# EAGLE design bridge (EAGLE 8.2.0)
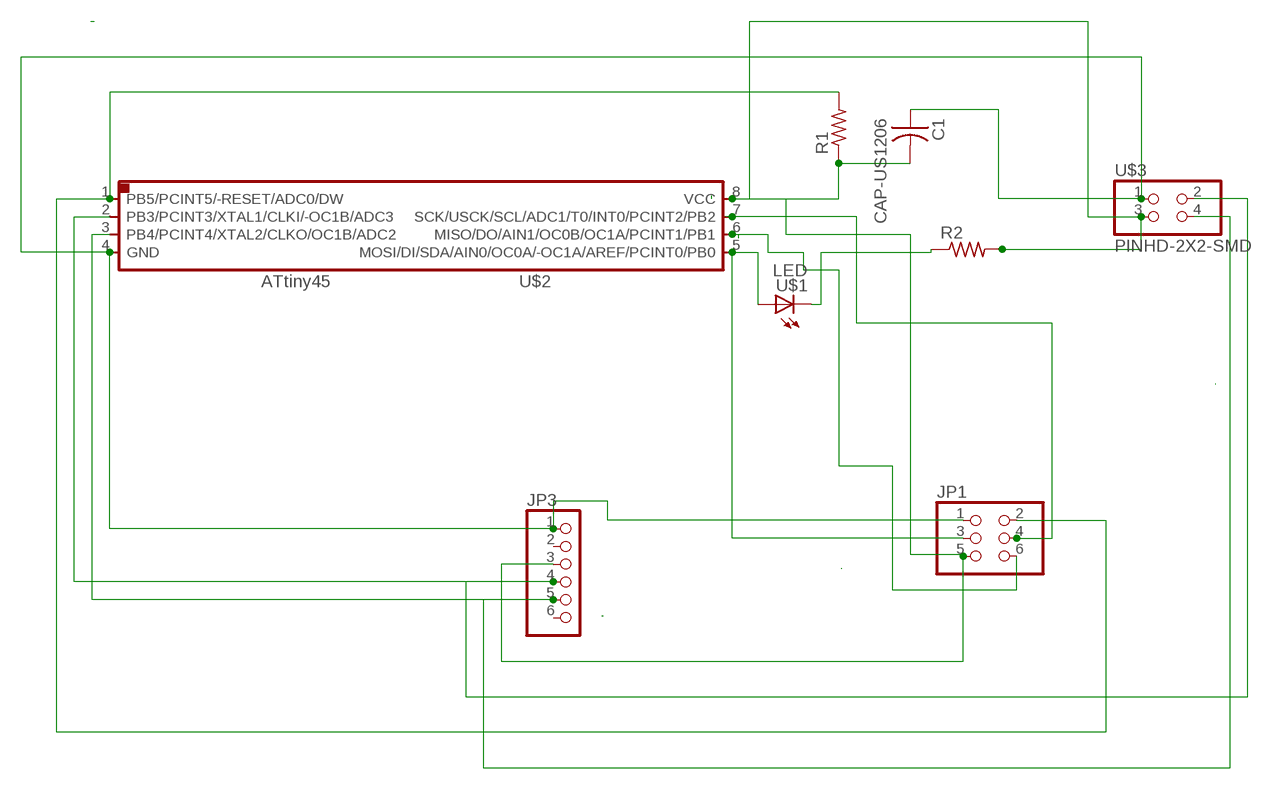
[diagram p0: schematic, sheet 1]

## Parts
C1  CAP-US1206  [C1206]
JP1  PINHD-2X3-SMD  [2X03SMD]
JP3  PINHD-1X6  [1X06]
R1  RES-US1206  [R1206]
R2  RES-US1206  [R1206]
U$1  LED  [LED1206]
U$2  ATTINY45SI  [SOIC8]
U$3  PINHD-2X2-SMD  [2X02SMD]

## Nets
N$2: JP1.6 U$2.6(MISO/DO/AIN1/OC0B/OC1A/PCINT1/PB1)
N$4: C1.1 JP1.1 JP3.1 U$2.4(GND) U$3.1
N$5: JP1.4 U$2.7(SCK/USCK/SCL/ADC1/T0/INT0/PCINT2/PB2)
N$6: JP3.4 U$2.2(PB3/PCINT3/XTAL1/CLKI/-OC1B/ADC3) U$3.2
N$7: JP3.5 U$2.3(PB4/PCINT4/XTAL2/CLKO/OC1B/ADC2) U$3.4
N$9: R2.1 U$1.2(C)
N$10: JP1.3 U$1.1(A) U$2.5(MOSI/DI/SDA/AIN0/OC0A/-OC1A/AREF/PCINT0/PB0)
N$12: JP1.2 R1.2 U$2.1(PB5/PCINT5/-RESET/ADC0/DW)
N$22: C1.2 JP1.5 JP3.3 R1.1 R2.2 U$2.8(VCC) U$3.3
Unconnected: JP3.2 JP3.6

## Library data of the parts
C1 = fab:CAP-US
JP1 = fab:PINHD-2X3-SMD: PIN HEADER
JP3 = pinhead:PINHD-1X6: PIN HEADER
R1 R2 = fab:RES-US: Resistor (US Symbol)
U$1 = fab:LED: LED
U$2 = fab:ATTINY45
U$3 = fab:PINHD-2X2-SMD

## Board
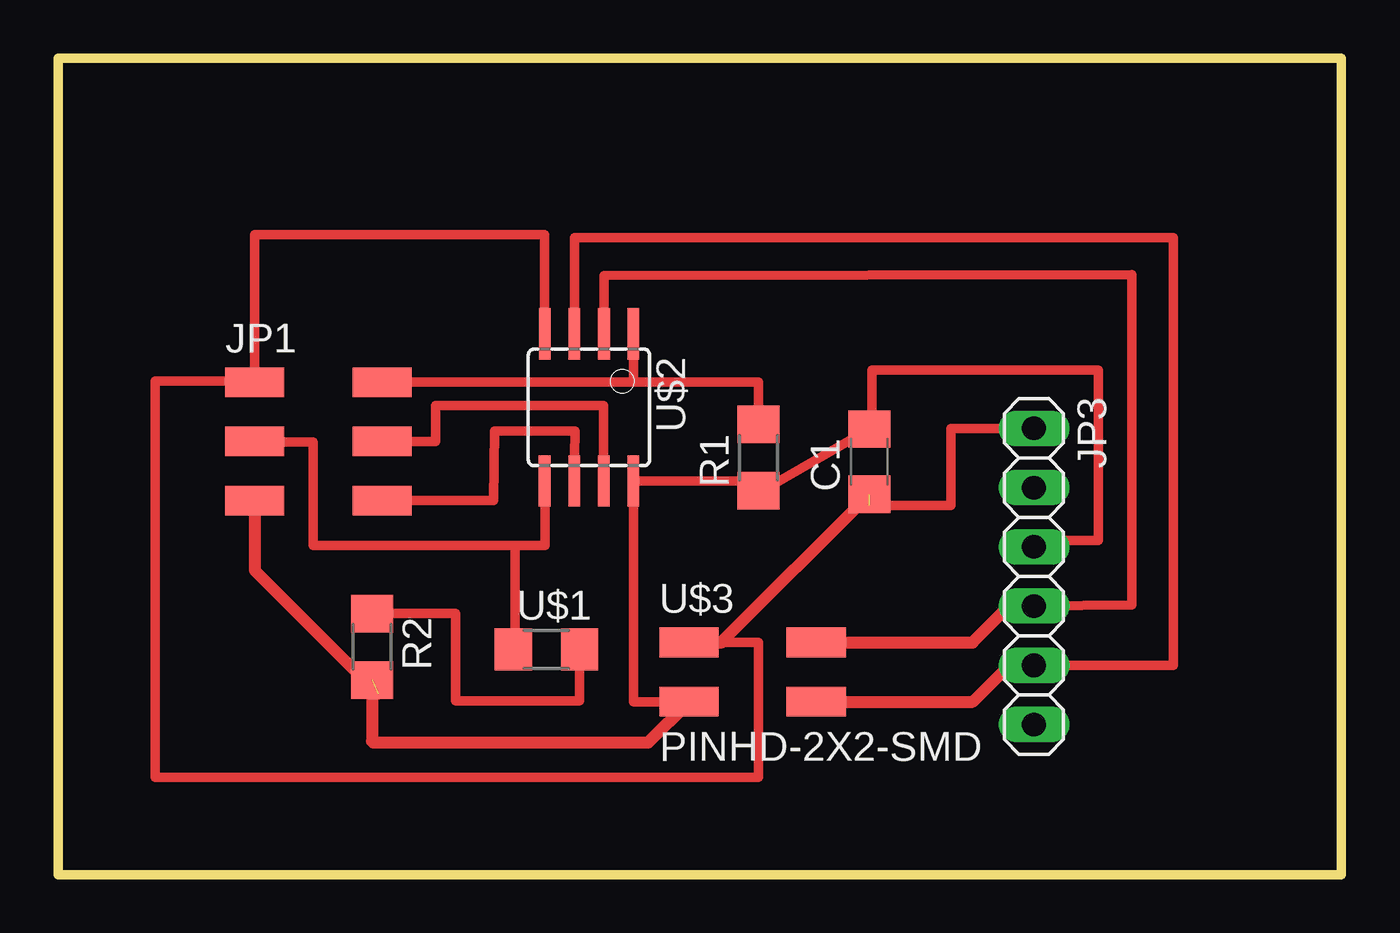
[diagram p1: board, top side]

Size 55 x 35 mm. Coordinates in mm from the lower left corner, seen from the top.
Outline: 0,35 0,0 55,0 55,35 0,35
Copper layers (1*16): Top 0.035mm / dielectric 1.5mm / Bottom 0.035mm
Design rules "default": minimum track width 10mil, minimum drill 24mil, track to track 8mil, track to pad 8mil, pad to pad 8mil, via to via 8mil, smd to smd 8mil, copper to edge 40mil, drill to drill 8mil, minimum pad ring 10mil, minimum via ring 8mil, stop-mask expansion 4mil, vias tented up to drill 0mil, thermal gap 10mil

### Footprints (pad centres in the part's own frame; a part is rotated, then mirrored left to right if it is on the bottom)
C1206 = smd 1.6 x 1.8: 1 -1.4,0; 2 1.4,0
2X03SMD = smd 2.54 x 1.27: 1 -2.54,2.54; 2 2.92,2.54; 3 -2.54,0; 4 2.92,0; 5 -2.54,-2.54; 6 2.92,-2.54
1X06 = drill 1.016 long: 1 -6.35,0; 2 -3.81,0; 3 -1.27,0; 4 1.27,0; 5 3.81,0; 6 6.35,0
R1206 = smd 1.6 x 1.803: 1 -1.422,0; 2 1.422,0
LED1206 = smd 1.6 x 1.803: 1 -1.422,0; 2 1.422,0
SOIC8 = smd 0.5 x 2.2: 1 -1.905,-3.154; 2 -0.645,-3.154; 3 0.625,-3.154; 4 1.895,-3.154; 5 1.905,3.154; 6 0.635,3.154; 7 -0.635,3.154; 8 -1.905,3.154
2X02SMD = smd 2.54 x 1.27: 1 -2.54,1.27; 2 2.92,1.27; 3 -2.54,-1.27; 4 2.92,-1.27

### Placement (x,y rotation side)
C1  34.77,17.7 90 top
JP1  10.96,18.57 0 top
JP3  41.83,12.78 270 top
R1  30.02,17.88 90 top
R2  13.45,9.76 270 top
U$1  20.92,9.66 0 top
U$2  22.75,20.03 180 top
U$3  29.58,8.68 0 top

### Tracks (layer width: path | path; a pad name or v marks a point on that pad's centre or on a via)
N$2
  Top 0.406: JP1.6 18.67,16.03 18.71,19.02 22.16,19.02 U$2.6
N$4  (1 unrouted)
  Top 0.406: U$2.4 20.86,27.44 8.42,27.44 8.42,24.39 JP1.1 8.42,21.17 4.15,21.17 4.15,4.16 30.02,4.16 30.02,9.95 U$3.1 | JP3.1 | 41.83,19.16 JP3.1 | C1.1 34.86,16.3 | JP3.1 38.26,19.13 38.26,15.84 34.77,15.84
  Top 0.508: U$3.1 28.42,9.95 C1.1
N$5
  Top 0.406: JP1.4 16.18,18.57 16.18,20.11 23.38,20.11 U$2.7
N$6
  Top 0.406: 32.97,9.95 U$3.2 | 41.83,12.08 JP3.4 46.02,11.55 46.02,25.71 23.39,25.67 U$2.2
  Top 0.508: U$3.2 39.19,9.95 40.62,11.38 41.7,11.38 JP3.4
N$7
  Top 0.406: 41.83,8.75 JP3.5 47.81,8.97 47.81,27.31 22.12,27.31 U$2.3
  Top 0.508: U$3.4 39.21,7.41 40.55,8.76 41.62,8.76 JP3.5
N$9
  Top 0.406: R2.1 17.03,11.19 17.03,7.45 22.34,7.45 U$1.2
N$10
  Top 0.406: 20.84,16.42 U$2.5 20.87,16.88 20.87,14.11 19.58,14.11 | 19.58,14.11 10.93,14.11 10.93,18.55 8.42,18.55 JP1.3 | U$1.1 19.58,9.66 19.58,14.11
N$12
  Top 0.406: U$2.1 24.65,23.69 | 24.65,23.38 U$2.1 | JP1.2 24.65,21.11 | 24.65,21.11 U$2.1 | 24.65,21.11 30.02,21.11 R1.2
N$22  (1 unrouted)
  Top 0.406: U$3.3 24.65,7.41 U$2.8 30.02,16.88 R1.1 30.02,16.35 C1.2 34.88,19.1 34.88,21.63 44.59,21.63 44.59,14.31 41.83,14.31 JP3.3 41.83,14.03
  Top 0.508: JP1.5 8.42,13.05 13.72,7.75 | R2.2 13.45,5.73 13.52,5.67 25.29,5.67 U$3.3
